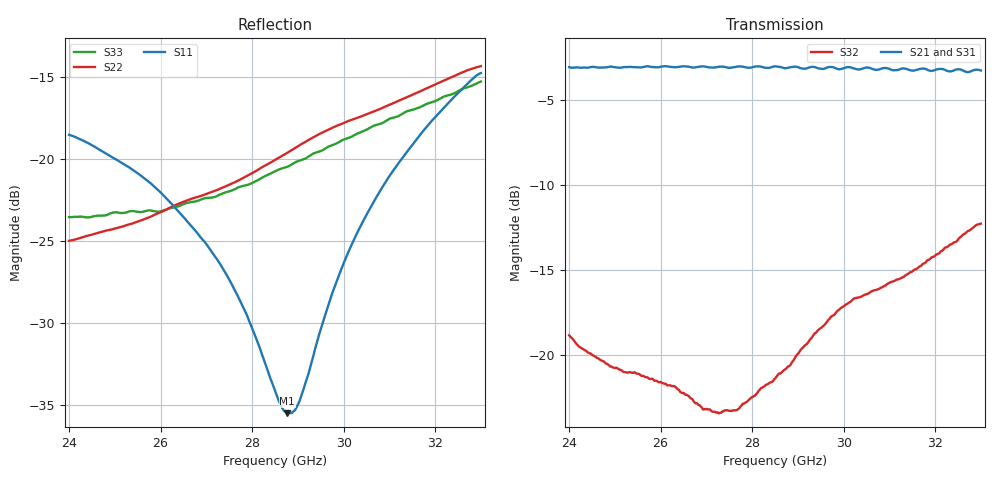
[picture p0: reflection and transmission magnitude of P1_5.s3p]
!The following data was pulled from an Agilent PNA
!This sNp file was generated from the data in the RF Test software
!NOTE:  Smoothing/Math/Corrections applied on any given trace ARE included in the data saved here
# MHz S dB R 50
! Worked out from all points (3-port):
!   1601 points, 24 GHz to 33 GHz, reference 50 ohm
!   strongest paths, dB at 24 GHz, 26.25 GHz, 28.5 GHz, 30.75 GHz, 33 GHz:
!     S21: -3.0, -3.0, -3.0, -3.2, -3.2
!     S31: -3.0, -3.0, -3.2, -3.2, -3.3
!     S32: -18.8, -21.8, -21.4, -16.1, -12.3
!   lowest |S11| = -35.5 dB at 28.76 GHz (marker M1), VSWR 1.03, Z = 49.9 - j1.68 ohm
!   |S11| at or under -10 dB: start of sweep to end of sweep
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24000  -18.51 27.7  -3.18 150.5  -3.15 150.5
       -3.05 150.3  -24.96 153.8  -18.82 80.2
       -3.02 149.9  -18.84 79.9  -23.52 171.2
25653.75  -21.17 9.7  -3.17 134.1  -3.15 134.1
          -3.02 134.1  -23.64 141.8  -21.29 46.0
          -3.03 133.4  -21.28 45.8  -23.16 155.7
26981.25  -25.10 -9.4  -3.06 120.5  -3.08 120.5
          -3.03 119.9  -22.13 133.7  -23.19 0.7
          -3.08 120.0  -23.20 0.5  -22.36 147.2
27780  -28.87 -25.8  -3.06 111.9  -3.11 112.0
       -3.02 111.7  -21.17 130.9  -22.90 -21.5
       -3.12 111.8  -22.92 -21.8  -21.63 142.9
28500  -34.11 -63.9  -3.07 104.4  -3.15 104.6
       -3.01 104.3  -20.03 127.9  -21.37 -44.4
       -3.17 104.3  -21.39 -44.4  -20.74 139.0
28764.38  -35.48 -92.2  -3.08 101.4  -3.17 101.7
          -3.10 101.6  -19.62 126.5  -20.72 -52.3
          -3.12 101.5  -20.73 -52.3  -20.45 137.4
29023.12  -34.81 -123.6  -3.06 98.6  -3.16 98.9
          -3.08 98.2  -19.16 125.0  -19.86 -59.0
          -3.17 99.2  -19.85 -59.1  -20.08 135.5
29799.38  -27.80 -173.9  -3.10 90.1  -3.18 90.8
          -3.08 90.0  -18.02 119.0  -17.62 -82.4
          -3.21 91.0  -17.63 -82.8  -19.08 129.7
30660  -22.58 166.8  -3.13 80.7  -3.19 81.6
       -3.18 80.7  -17.08 112.7  -16.17 -104.8
       -3.19 82.0  -16.19 -105.0  -17.95 122.8
33000  -14.74 134.6  -3.36 54.4  -3.34 55.6
       -3.25 54.9  -14.32 97.1  -12.20 -143.6
       -3.29 56.3  -12.27 -143.8  -15.25 101.7
